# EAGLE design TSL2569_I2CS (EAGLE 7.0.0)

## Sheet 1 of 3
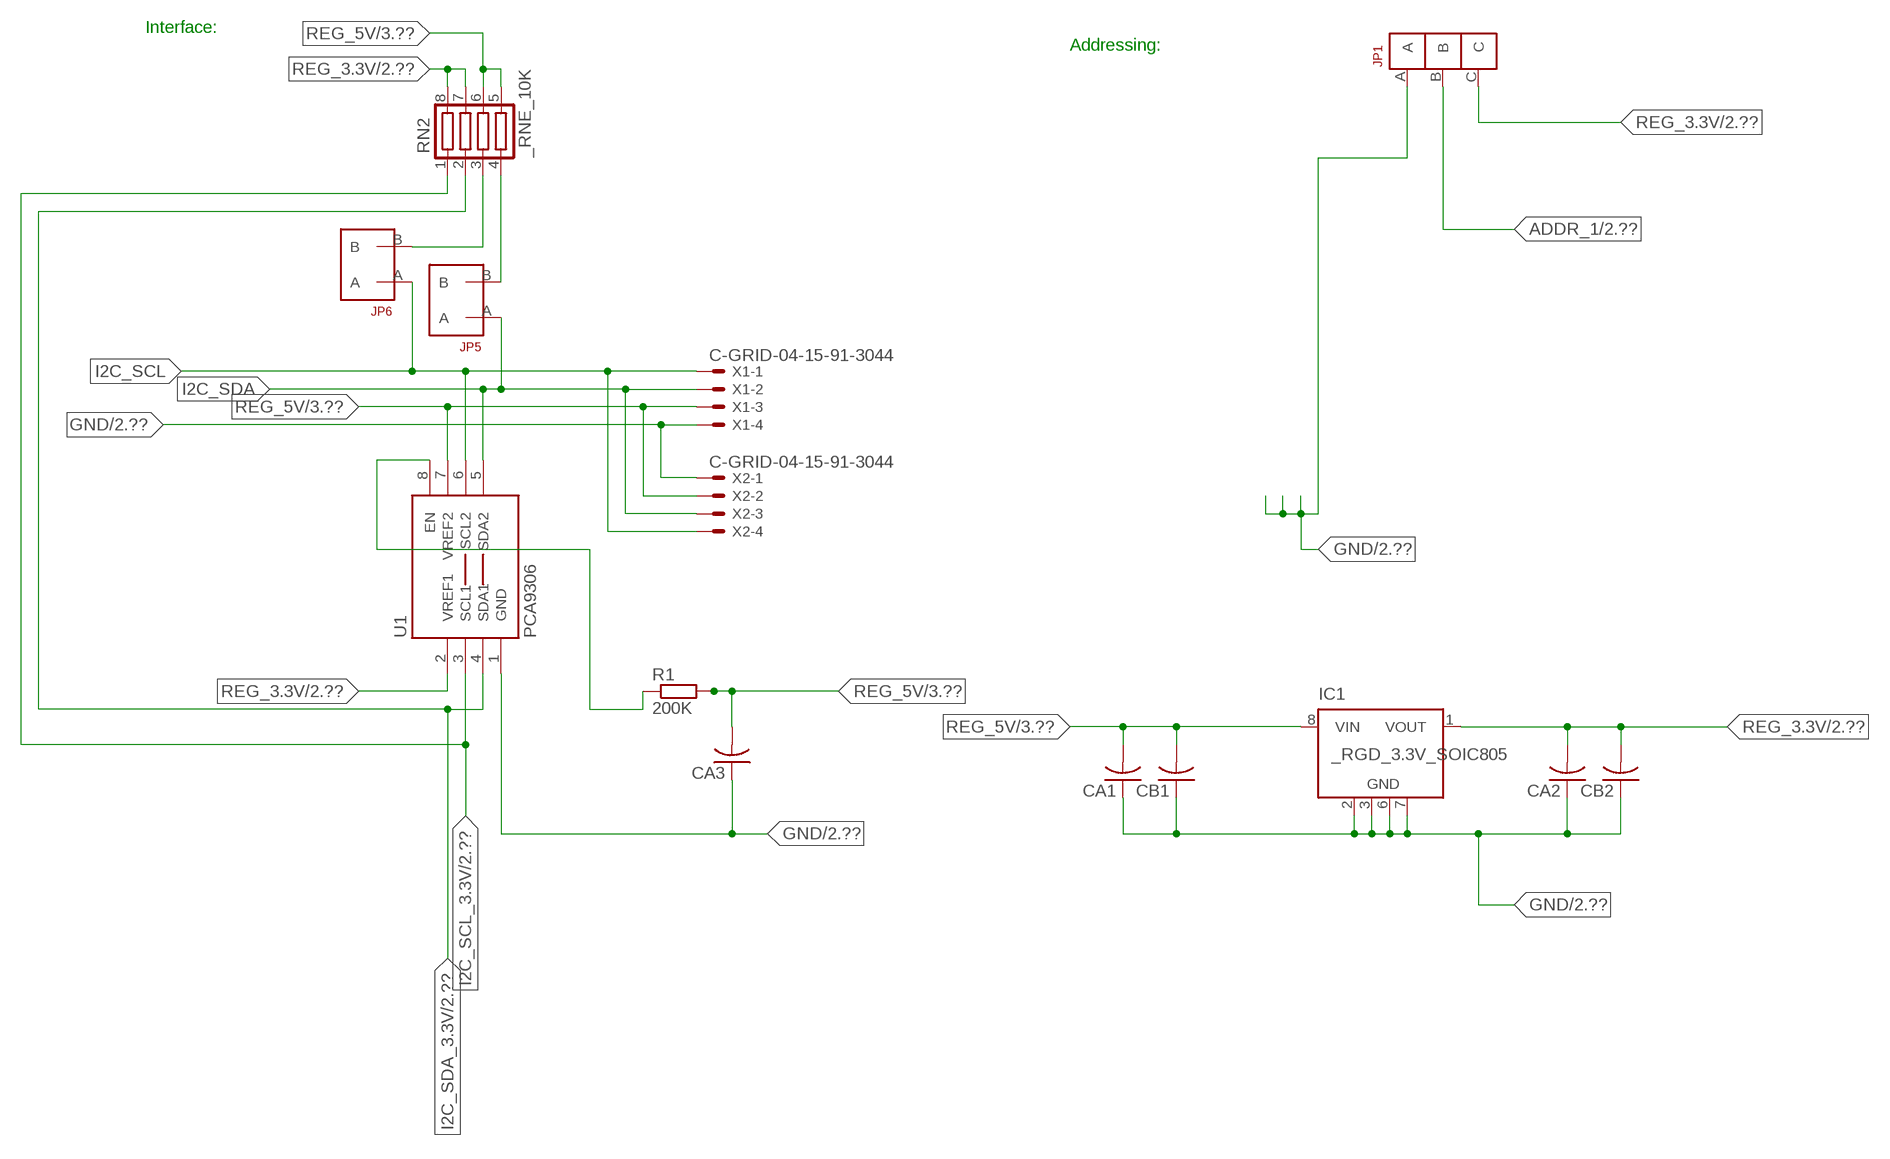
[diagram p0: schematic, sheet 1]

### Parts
CA1  CC1206KRX7R9BB104  [.1UF]
CA2  CC1206KRX7R9BB104  [.1UF]
CA3  CC1206KRX7R9BB104  [.1UF]
CB1  TMK316F106ZL-TC1206K  [TMK316F106ZL-T]
CB2  TMK316F106ZL-TC1206K  [TMK316F106ZL-T]
IC1  _RGD_3.3V_SOIC805  [_RGC_3.3V_SOIC8]
JP1  JUMPER_1X3_2MM  [JUMPER_1X3_2MM]
JP5  JUMPER_1X2_2MM  [JUMPER_1X2_2MM]
JP6  JUMPER_1X2_2MM  [JUMPER_1X2_2MM]
R1  200K  RESISTOR_SMT-0603  [R603]
RN2  _RNE_10K  [RNE]
U1  PCA9306  PCA9306_NCD  [PSOP-8]
X1  C-GRID-04-15-91-3044  [15-91-04]
X2  C-GRID-04-15-91-3044  [15-91-04]

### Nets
ADDR_1: JP1.B ; also sheet 2
GND: CA1.1 CA2.1 CA3.1 CB1.1 CB2.1 IC1.2(GND) IC1.3(GND) IC1.6(GND) IC1.7(GND) JP1.A U1.1(GND) X1.4 X2.1 ; also sheet 2,3
I2C_SCL: JP6.A U1.6(SCL2) X1.1 X2.4
I2C_SCL_3.3V: RN2.1 U1.3(SCL1) ; also sheet 2
I2C_SDA: JP5.A U1.5(SDA2) X1.2 X2.3
I2C_SDA_3.3V: RN2.2 U1.4(SDA1) ; also sheet 2
N$1: JP6.B RN2.3
N$2: JP5.B RN2.4
N$23: R1.1 U1.8(EN)
REG_3.3V: CA2.2 CB2.2 IC1.1(VOUT) JP1.C RN2.7 RN2.8 U1.2(VREF1) ; also sheet 2
REG_5V: CA1.2 CA3.2 CB1.2 IC1.8(VIN) R1.2 RN2.5 RN2.6 U1.7(VREF2) X1.3 X2.2 ; also sheet 3
Unconnected: IC1.4(NC) IC1.5(NC)

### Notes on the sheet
- Interface:
- Addressing:

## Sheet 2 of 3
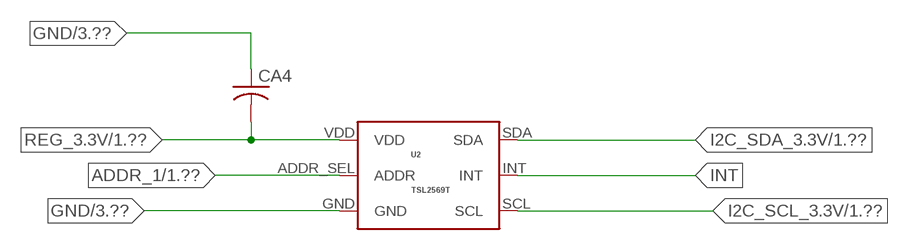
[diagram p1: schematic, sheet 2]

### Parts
CA4  _CA_.10UF_50VC1206K  [_CA_.1UF_50V]
U2  TSL2569T  TSL2561T  [TSL2561T]

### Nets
ADDR_1: U2.ADDR_SEL(ADDR) ; also sheet 1
GND: CA4.1 U2.GND ; also sheet 1,3
I2C_SCL_3.3V: U2.SCL ; also sheet 1
I2C_SDA_3.3V: U2.SDA ; also sheet 1
INT: U2.INT
REG_3.3V: CA4.2 U2.VDD ; also sheet 1

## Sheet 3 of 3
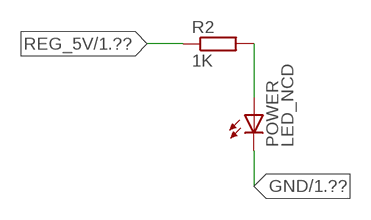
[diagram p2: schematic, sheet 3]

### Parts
POWER  LED_NCD  [CHIPLED_0603]
R2  1K  RESISTOR_SMT-0402  [R402]

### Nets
GND: POWER.C ; also sheet 1,2
N$4: POWER.A R2.2
REG_5V: R2.1 ; also sheet 1

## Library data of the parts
CA1-CA3 = NCD_ULTIMATE_LIBRARY:CC1206KRX7R9BB104: Capacitor CA .1uF 50V SMT C1206K CC1206KRX7R9BB104
CA4 = NCD_ULTIMATE_LIBRARY:_CA_.10UF_50V: Capacitor .1uF SMT
CB1 CB2 = NCD_ULTIMATE_LIBRARY:TMK316F106ZL-T: Capacitor CB 10uF SMT 1206 TMK316F106ZL-T
IC1 = NCD_ULTIMATE_LIBRARY:_RGD_3.3V_SOIC8: Regulator Linear 3.3V Chip Positive VOLTAGE REGULATOR Digikey 497-1199-2-ND/L78L33ACD13TR
JP1 = NCD_ULTIMATE_CONNECTORS:JUMPER_1X3_2MM
JP5 JP6 = NCD_ULTIMATE_CONNECTORS:JUMPER_1X2_2MM
POWER = NCD_ULTIMATE_LIBRARY:LED_NCD: LED Digikey 754-1132-2-ND/APT2012SRCPRV
R1 R2 = NCD_ULTIMATE_LIBRARY:RESISTOR_SMT: NCD Resistor
RN2 = NCD_ULTIMATE_LIBRARY:_RNE_10K: Resistor Array RNE SMT 10K x 4 Single Resistor Source: http://www.ctscorp.com/components/Datasheets/CTSChipArrayDs.pdf Digikey 742C083103JPTR-ND/742C083103JP; OC_FARNELL: unknown; OC_NEWARK: unknown
U1 = NCD_ULTIMATE_LIBRARY:PCA9306_NCD: NCD Bidirectional I2C level shifter. NOT compatible with all available part number pinout schemes- DOUBLE CHECK!!!; PROD_ID: IC-10023
U2 = NCD_ULTIMATE_bhaskar:TSL2561T: Digikey TSL2569-TDKR-ND/TSL2569T
X1 X2 = NCD_ULTIMATE_CONNECTORS:C-GRID-04: CONNECTOR 4-Pos I2C wire to board 2.54 mm (0.100") pitch header Digikey WM1342-ND/0015912045; OC_FARNELL: unknown; OC_NEWARK: unknown

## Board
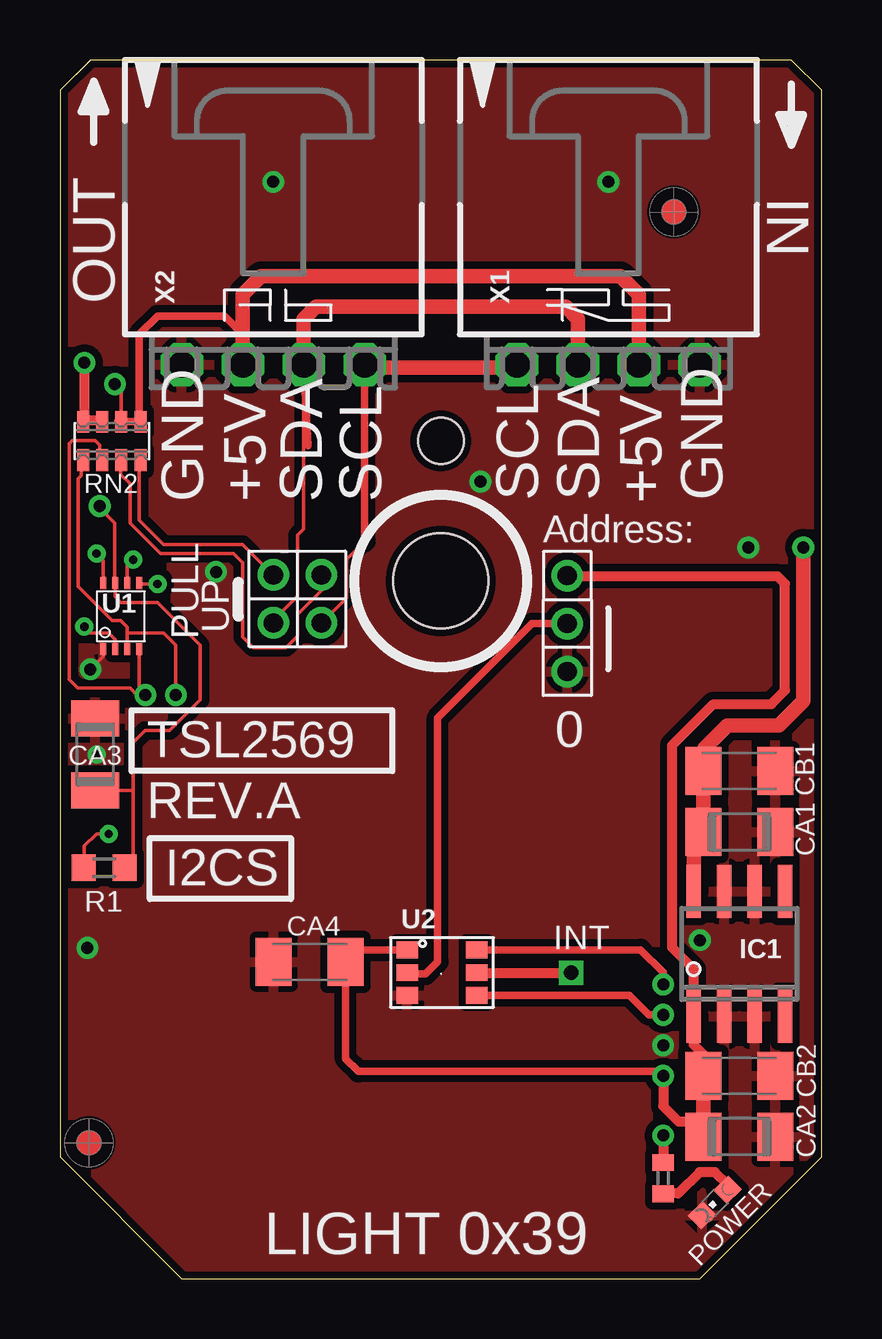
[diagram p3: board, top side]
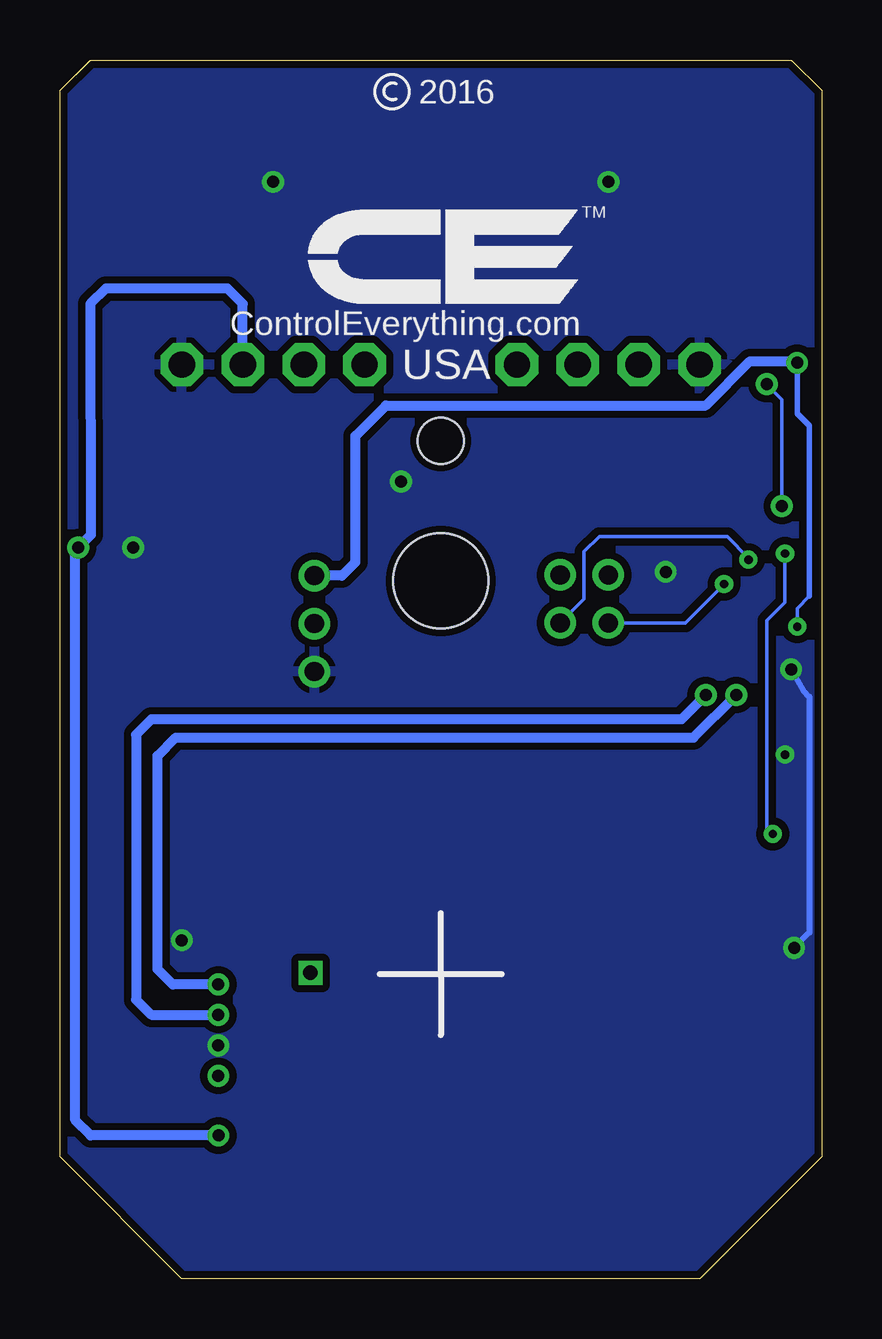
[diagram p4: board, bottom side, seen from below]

Size 31.75 x 50.8 mm. Coordinates in mm from the lower left corner, seen from the top.
Outline: 32 segments
Copper layers (1*16): Top 0.035mm / dielectric 1.5mm / Bottom 0.035mm
Design rules "default": minimum track width 5mil, minimum drill 24mil, track to track 5mil, track to pad 5mil, pad to pad 5mil, via to via 5mil, smd to smd 5mil, copper to edge 10mil, drill to drill 8mil, minimum pad ring 10mil, minimum via ring 8mil, stop-mask expansion 2mil, vias tented up to drill 0mil, thermal gap 10mil
Holes 3.96 mm at 15.88,29.08
Holes 1.91 mm at 15.88,34.93

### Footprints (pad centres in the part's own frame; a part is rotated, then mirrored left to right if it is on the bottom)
.1UF = smd 1.5 x 2: 1 -1.5,0; 2 1.5,0
_CA_.1UF_50V = smd 1.5 x 2: 1 -1.5,0; 2 1.5,0
TMK316F106ZL-T = smd 1.5 x 2: 1 -1.5,0; 2 1.5,0
_RGC_3.3V_SOIC8 = smd 0.6 x 2.2: 1 -1.905,-2.6; 2 -0.635,-2.6; 3 0.635,-2.6; 4 1.905,-2.6; 5 1.905,2.6; 6 0.635,2.6; 7 -0.635,2.6; 8 -1.905,2.6
JUMPER_1X3_2MM = drill 0.8: A 0,2; B 0,0; C 0,-2
JUMPER_1X2_2MM = drill 0.8: A 0,2; B 0,0
CHIPLED_0603 = smd 0.8 x 0.876: A 0,-0.75; C 0,0.75
R603 = smd 1 x 1.1: 1 -0.85,0; 2 0.85,0
R402 = smd 0.7 x 0.9: 1 -0.65,0; 2 0.65,0
RNE = smd 0.5 x 0.9: 1 -1.2,-0.8; 2 -0.4,-0.8; 3 0.4,-0.8; 4 1.2,-0.8; 5 1.2,0.8; 6 0.4,0.8; 7 -0.4,0.8; 8 -1.2,0.8
PSOP-8 = smd 0.25 x 0.5: 1 -0.73,-1.37; 2 -0.23,-1.37; 3 0.27,-1.37; 4 0.77,-1.37; 5 0.77,1.38; 6 0.27,1.38; 7 -0.23,1.38; 8 -0.73,1.38
TSL2561T = smd 0.9 x 0.7: ADDR_SEL 0,0.95; GND 0,0; INT 2.9,0.95; SCL 2.9,0; SDA 2.9,1.9; VDD 0,1.9
15-91-04 = drill 1.1 pad 1.778 octagon: 1 -3.81,-7.62; 2 -1.27,-7.62; 3 1.27,-7.62; 4 3.81,-7.62

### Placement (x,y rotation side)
CA1  28.32,18.62 180 top
CA2  28.32,5.92 180 top
CA3  1.46,21.86 270 top
CA4  10.41,13.21 0 top
CB1  28.32,21.16 180 top
CB2  28.32,8.46 180 top
IC1  28.32,13.54 0 top
JP1  21.15,27.31 180 top
JP5  8.89,29.34 180 top
JP6  10.9,29.34 180 top
POWER  27.3,3.18 135 top
R1  1.84,17.13 0 top
R2  25.15,4.19 270 top
RN2  2.16,34.93 0 top
U1  2.54,27.61 0 top
U2  14.48,11.81 0 top
U$5  [VISION_REF10]  1.21,5.66 90 top
U$28  [VISION_REF10]  25.59,44.46 90 top
X1  22.86,45.72 0 top
X2  8.89,45.72 0 top

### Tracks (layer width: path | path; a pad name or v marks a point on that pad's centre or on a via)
ADDR_1
  Top 0.305: U2.ADDR_SEL 14.54,12.7 15.24,12.7 15.75,13.21 15.75,23.37 19.68,27.31 JP1.B
GND  (via drill 0.35, 0.5)
  Top 0.152: CA3.1 1.52,23.42 1.52,23.62 | v1.27,25.4 1.81,25.94 U1.1
  Bottom 0.254: v1.27,25.4 0.76,24.51 0.51,24.26 0.51,14.43 v1.15,13.79
  other vias: 8.89,45.72 22.86,45.72 25.15,9.73 17.53,33.22 26.67,14.11 6.5,29.46 28.7,30.48 1.52,21.84
  pour Bottom (isolate 0.305): -0.64,5.08 -0.64,49.53 1.27,51.44 30.48,51.44 32.38,49.53 32.38,5.08 26.67,-0.63 5.08,-0.63
  pour Top (isolate 0.305): 4.45,-1.27 -1.27,4.45 -1.27,50.17 0.64,52.07 31.11,52.07 33.02,50.17 33.02,4.45 27.3,-1.27
I2C_SCL  (via drill 0.35)
  Top 0.152: 12.7,30.73 11.94,29.97 11.94,28.38 JP6.A | v3.05,29.97 2.81,29.73 U1.6
  Top 0.305: 12.7,30.73 X2.4
  Top 0.406: X2.4 12.7,37.97 | 19.05,37.97 X1.1
  Top 0.61: 12.7,37.97 19.05,37.97
  Bottom 0.152: JP6.A 9.91,28.33 9.91,30.3 9.27,30.94 3.94,30.94 3.05,30.05 v3.05,29.97
I2C_SCL_3.3V  (via drill 0.5)
  Top 0.152: RN2.1 0.89,34.07 0.89,33.48 0.77,33.35 0.77,28.84 2.17,27.43 2.54,27.43 2.81,27.17 2.81,26.92 | 2.81,26.92 U1.3 | v4.83,24.33 v4.83,24.34 4.83,26.42 4.32,26.92 2.81,26.92
  Top 0.305: U2.SCL 23.75,11.81 24.56,11 v25.15,11
  Bottom 0.406: v4.83,24.33 5.84,23.32 27.94,23.32 28.58,22.68 28.58,11.63 27.94,11 v25.15,11
I2C_SDA  (via drill 0.35)
  Top 0.152: JP5.A 8.89,27.44 9.91,28.45 9.91,30.99 10.16,31.24 10.16,34.92 X2.3 | U1.5 3.34,28.96 v4.06,28.96
  Top 0.305: 10.35,34.73 X2.3
  Top 0.61: X2.3 10.16,40.01 10.67,40.51 21.09,40.51 21.59,40.01 X1.2
  Bottom 0.152: v4.06,28.96 5.68,27.34 JP5.A
I2C_SDA_3.3V  (via drill 0.5)
  Top 0.152: RN2.2 1.65,34.14 1.65,34.75 1.46,34.94 0.51,34.94 0.38,34.81 0.38,26.37 0.38,26.36 0.38,24.97 0.74,24.61 2.92,24.61 3.2,24.33 v3.56,24.33 3.31,24.58 U1.4
  Top 0.305: U2.SDA 17.26,13.72 24.21,13.72 25.15,12.77 v25.15,12.27
  Bottom 0.406: v25.15,12.27 27.05,12.27 27.69,12.9 27.69,21.79 26.93,22.56 5.34,22.56 v3.56,24.33
INT  (via drill 0.6)
  Top 0.406: U2.INT 17.26,12.75 v21.31,12.75
N$1
  Top 0.152: JP6.B 10.92,29.31 10.92,28.7 9.91,27.69 9.91,26.8 9.42,26.31 8.06,26.31 7.62,26.75 7.62,29.84 7.24,30.23 4.19,30.23 2.92,31.5 2.92,33.15 2.54,33.53 2.54,34.1 RN2.3
  Top 0.305: 2.54,34.02 RN2.3
N$2
  Top 0.152: JP5.B 7.62,30.61 4.32,30.61 3.3,31.62 3.3,34.07 RN2.4
  Top 0.305: 3.37,33.88 RN2.4
N$4
  Top 0.406: POWER.A 27.84,3.92 27.3,4.45 26.67,4.45 25.78,3.56 25.16,3.56 R2.2
N$23  (via drill 0.35)
  Top 0.152: R1.1 1.02,17.16 1.02,18.03 1.52,18.54 v2.03,18.54 | v1.52,30.23 1.81,29.94 U1.8
  Bottom 0.152: v2.03,18.54 2.29,18.8 2.29,27.43 1.52,28.19 v1.52,30.23
REG_3.3V  (via drill 0.35, 0.5)
  Top 0.152: v1.02,27.18 1.27,26.92 2.03,26.92 2.31,26.65 U1.2
  Top 0.305: U2.VDD 12.29,13.71 CA4.2 11.91,9.17 12.45,8.64 24.89,8.64 25.15,8.38 25.15,7.19
  Top 0.406: CB2.2 26.82,9.35 26.42,9.75 26.42,10.36 | v25.15,8.46 25.15,7.19 25.78,6.55 26.82,6.55 | IC1.1 26.42,12.9 25.53,13.79 25.53,22.24 27.24,23.95 29.66,23.95 30.23,24.52 30.23,28.97 29.91,29.29 21.17,29.29 JP1.C | 26.52,5.62 CA2.2 | v1.02,38.18 1.02,35.78 | 1.02,35.78 RN2.8 | 1.02,35.78 1.71,35.78 RN2.7
  Top 0.61: CB2.2 26.82,6.55 CA2.2 | 26.42,10.36 IC1.1
  Bottom 0.152: 0.51,28.45 1.02,27.94 v1.02,27.18
  Bottom 0.229: 0.51,28.45 0.51,35.56 1.02,36.07 v1.02,38.18
  Bottom 0.406: v1.02,38.18 1.08,38.24 2.99,38.24 4.83,36.4 18.16,36.4 19.43,35.13 19.43,29.87 20,29.31 JP1.C
REG_5V  (via drill 0.5)
  Top 0.152: RN2.6 2.56,37.01 v2.29,37.29 | R1.2 3.05,17.49 3.05,20.36 | 3.05,20.36 3.05,22.35 3.56,22.86 4.57,22.86 5.84,24.13 5.84,26.42 4.06,28.19 2.54,28.19 2.31,28.43 U1.7 2.29,29.01 2.29,31.5 1.65,32.13 v1.65,32.21 | CA3.2 3.05,20.36
  Top 0.305: 7.62,39.37 7.5,39.37 | 2.42,35.74 RN2.6 RN2.5 3.31,35.8 3.31,39.37 4.07,40.13 6.86,40.13 7.62,39.37 | X2.2 7.62,39.37
  Top 0.406: v25.15,5.97 R2.1
  Top 0.61: X1.3 24.13,41.02 23.37,41.78 8.38,41.78 7.62,41.02 X2.2 | IC1.8 26.42,18.21 CA1.2 CB1.2 26.86,21.2 26.86,22.11 27.82,23.06 29.98,23.06 30.99,24.08 v30.99,30.48
  Bottom 0.152: v1.65,32.21 1.65,36.65 v2.29,37.29
  Bottom 0.406: X1.3 24.13,40.64 24.77,41.28 29.84,41.28 30.48,40.64 30.47,31 v30.99,30.48 31.11,30.36 31.11,6.6 30.48,5.97 v25.15,5.97

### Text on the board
tPlace: LIGHT 0x39
tNames: IN | OUT | GND | +5V | SDA | SCL | SCL | SDA | +5V | GND | Address: | PULL | UP | TSL2569 | 0 | REV.A | I2CS | INT
bNames: 2016 | TM | ControlEverything.com | USA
